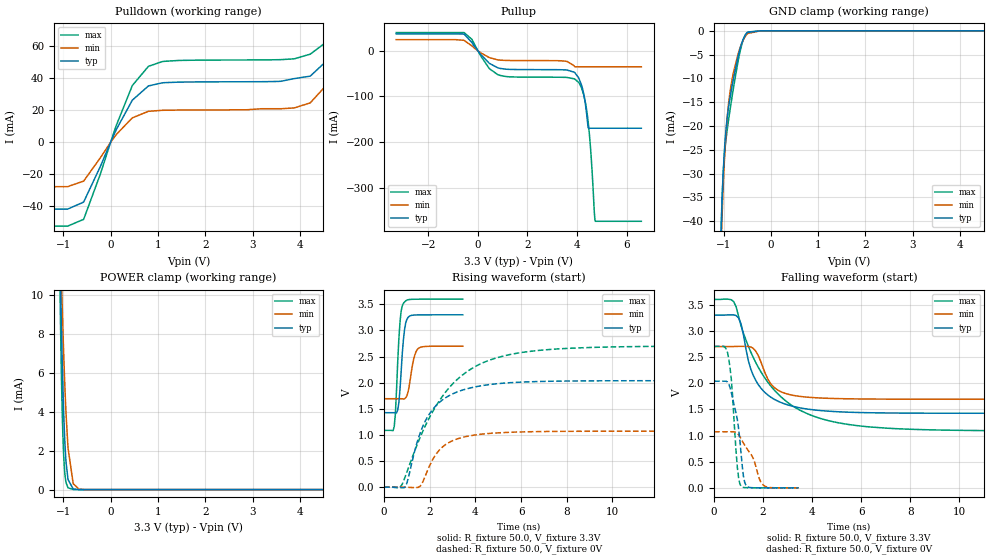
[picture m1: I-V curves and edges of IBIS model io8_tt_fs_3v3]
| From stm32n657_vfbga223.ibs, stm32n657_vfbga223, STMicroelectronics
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[Model]   io8_tt_fs_3v3
Model_type I/O
Polarity   Non-Inverting
Enable   Active-Low
| CAP_THRESHOLD on pad IOTT is "UDTCAPC" :
| Rising=30.0% of vddiov33m   Falling=70.0% of vddiov33m
| C_comp min and max val. don't necessarily correlate with the min and max pvt
| but are the smallest and greatest pad capacitance found.
| var   typ   min   max
C_comp   1.01876pF  1.01074pF  1.02142pF
|C_comp_pullup   495.66000fF  479.36000fF  510.70500fF
|C_comp_pulldown   523.10000fF  531.38429fF  510.71500fF
Vinl = 1.35V
Vinh = 1.8V
Vmeas = 1.65V   | Reference voltage for timing measurements
Cref  = 50.0pF   | Timing specification test load capacitance value
Rref  = 1.0MOhm   | Timing specification test load resistance value
Vref  = 1.815V   | Timing specification test load voltage
[Model Spec]
| TIME_THRESHOLD on pin ZIV08M is "CMOS" :
| Rising=50.0% of vddv08m   Falling=50.0% of vddv08m
Vinl 1.08570V 868.70000mV 1.21270V
Vinh 1.55630V 1.26230V 1.70930V
| variable   typ   min   max
[Temperature Range] 25.0 125.0 -40.0
| variable   typ   min   max
[Voltage Range] 3.3V 2.7V 3.6V
| variable   typ   min   max
[POWER Clamp Reference] 3.3V 2.7V 3.6V
| variable   typ   min   max
[GND Clamp Reference] 0V 0V 0V
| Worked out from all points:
|   slope of the pulldown table from 0 to 0.495 V, typ, clamps not added: 18.2 ohm
|   slope of the pullup table from 0 to 0.495 V, typ, clamps not added: 17.3 ohm
|   GND clamp passes 1 mA (typ) near -0.55 V on its own axis
|   POWER clamp passes 1 mA (typ) near -0.92 V on its own axis
|   rising waveform, R_fixture 50.0, V_fixture 3.3V: 20-80 % time 190ps typ, 243ps min, 172ps max; typ from 1.43 V to 3.3 V
|   falling waveform, R_fixture 50.0, V_fixture 3.3V: 20-80 % time 929ps typ, 690ps min, 2.03ns max; typ from 3.3 V to 1.43 V
|   rising waveform, R_fixture 50.0, V_fixture 0V: 20-80 % time 1.26ns typ, 1.05ns min, 2.27ns max; typ from 0 V to 2.04 V
|   falling waveform, R_fixture 50.0, V_fixture 0V: 20-80 % time 355ps typ, 624ps min, 240ps max; typ from 2.04 V to 0 V
[POWER Clamp]
-3.3V     1.353A     318.4mA    2.015A
-1.07V    12.07mA    13.62mA    10.38mA
-1.06V    10.79mA    12.68mA    8.745mA
-1.05V    9.571mA    11.76mA    7.253mA
-1.03V    7.341mA    9.999mA    4.748mA
-1V       4.588mA    7.595mA    2.215mA
-980mV    3.183mA    6.171mA    1.238mA
-950mV    1.704mA    4.337mA    481.8uA
-900mV    515.5uA    2.141mA    93.34uA
-790mV    29.45uA    301.7uA    4.884uA
-670mV    1.871uA    28.97uA    2.19uA
6.6V      0A         0A         0A
[GND Clamp]
-3.3V     -3.772A    -3.743A    -3.788A
-1.05V    -42.34mA   -45.44mA   -41.2mA
-1.04V    -38.9mA    -42mA      -37.88mA
-1.03V    -35.84mA   -38.88mA   -35.06mA
-1V       -28.57mA   -31.07mA   -28.88mA
-970mV    -23.48mA   -25.09mA   -24.97mA
-920mV    -18.07mA   -17.99mA   -20.63mA
-860mV    -13.91mA   -12.68mA   -16.46mA
-780mV    -9.536mA   -8.318mA   -11.38mA
-650mV    -3.744mA   -3.567mA   -4.327mA
-490mV    -324.2uA   -555.2uA   -259.7uA
6.6V      214nA      4.276uA    223.3nA
| variable   typ   min   max
[Pullup Reference] 3.3V 2.7V 3.6V
| variable   typ   min   max
[Pulldown Reference] 0V 0V 0V
[Pullup]
-3.3V     37.13mA    24.46mA    39.98mA
-560mV    36.73mA    22.97mA    39.98mA
800mV     -37.34mA   -19.93mA   -52.27mA
3.53V     -41.95mA   -22.74mA   -58.3mA
3.91V     -47.9mA    -35.06mA   -62.17mA
4.2V      -78.22mA   -35.06mA   -84.3mA
4.39V     -138.2mA   -35.06mA   -130mA
4.45V     -167.6mA   -35.06mA   -155.6mA
4.54V     -169.9mA   -35.06mA   -208.7mA
4.7V      -169.9mA   -35.06mA   -353.6mA
4.74V     -169.9mA   -35.06mA   -374mA
6.6V      -169.9mA   -35.06mA   -374mA
[Pulldown]
-3.3V     -41.68mA   -27.67mA   -52.26mA
-910mV    -41.66mA   -27.66mA   -52.26mA
-570mV    -37.25mA   -24.18mA   -48.03mA
120mV     7.91mA     4.86mA     10.53mA
460mV     26.3mA     15.25mA    35.41mA
800mV     35.13mA    19.32mA    47.35mA
1.43V     37.49mA    20.09mA    50.99mA
3.88V     39.68mA    21.4mA     52mA
4.22V     41.24mA    24.57mA    54.93mA
4.56V     50.57mA    35.57mA    62.45mA
4.9V      81.48mA    69.85mA    90.32mA
6.6V      932.4mA    945.7mA    856.3mA
[Ramp]
dV/dt_r 1.22272V/1.25681ns 642.93747mV/1.04416ns 1.62249V/2.27334ns
dV/dt_f 1.12484V/926.81681ps 604.28703mV/685.318ps 1.50794V/2.02571ns
R_load = 50.0
| Removed startup time: 0s 0s 0s  .
| Removed end time: 3.45ns.
[Rising Waveform]
R_fixture   = 50.0
V_fixture   = 3.3V
V_fixture_min = 2.7V
V_fixture_max = 3.6V
0s        1.425V     1.693V     1.087V
450ps     1.425V     1.693V     1.159V
500ps     1.424V     1.693V     1.402V
600ps     1.473V     1.693V     2.375V
700ps     1.86V      1.693V     3.145V
850ps     2.813V     1.688V     3.516V
1.05ns    3.247V     1.815V     3.587V
1.3ns     3.294V     2.45V      3.597V
1.5ns     3.298V     2.655V     3.598V
3.45ns    3.3V       2.7V       3.6V
| Removed startup time: 0s 0s 0s  .
| Removed end time: 24.9ns.
[Falling Waveform]
R_fixture   = 50.0
V_fixture   = 3.3V
V_fixture_min = 2.7V
V_fixture_max = 3.6V
0s        3.3V       2.7V       3.6V
700ps     3.305V     2.7V       3.594V
1ns       3.245V     2.704V     3.275V
1.5ns     2.266V     2.691V     2.592V
1.8ns     1.975V     2.529V     2.306V
2.2ns     1.771V     2.072V     2.014V
3ns       1.585V     1.792V     1.632V
4.9ns     1.458V     1.707V     1.26V
9.1ns     1.426V     1.693V     1.106V
24.9ns    1.425V     1.693V     1.087V
| Removed startup time: 0s 0s 0s  .
| Removed end time: 24.9ns.
[Rising Waveform]
R_fixture   = 50.0
V_fixture   = 0V
V_fixture_min = 0V
V_fixture_max = 0V
0s        357.9nV    2.11uV     435.7nV
700ps     -8.376mV   -125.3uV   -7.467mV
900ps     -7.517mV   -1.778mV   163.5mV
1.5ns     927.9mV    -4.415mV   864.9mV
1.7ns     1.164V     100.7mV    1.069V
2.4ns     1.613V     698.4mV    1.637V
3.7ns     1.89V      978mV      2.231V
5.3ns     1.993V     1.046V     2.518V
10ns      2.036V     1.071V     2.684V
24.9ns    2.038V     1.072V     2.704V
| Removed startup time: 0s 0s 0s  .
| Removed end time: 3.45ns.
[Falling Waveform]
R_fixture   = 50.0
V_fixture   = 0V
V_fixture_min = 0V
V_fixture_max = 0V
0s        2.038V     1.072V     2.704V
400ps     2.038V     1.072V     2.702V
550ps     2.022V     1.072V     2.583V
700ps     1.827V     1.072V     2.095V
950ps     1.301V     1.042V     390.9mV
1.1ns     663.9mV    939.6mV    30.43mV
1.2ns     217mV      853.2mV    8.358mV
1.35ns    24.42mV    741.7mV    3.111mV
2ns       865.4uV    56.77mV    857uV
3.45ns    207.1uV    263.7uV    235.3uV
